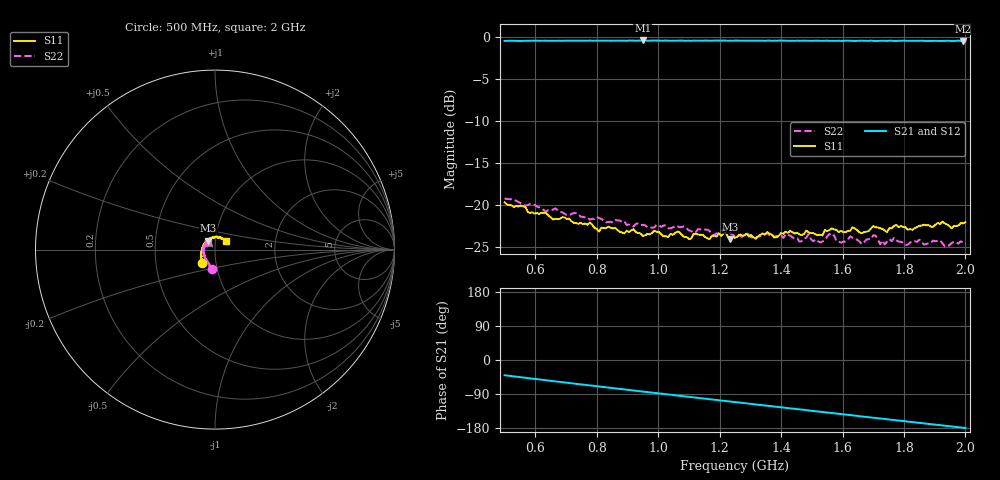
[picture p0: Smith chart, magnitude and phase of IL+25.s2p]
!Agilent Technologies,E8361C,US49010292,A.09.42.06
!Agilent E8361C: A.09.42.06
!Date: Friday, January 10, 2025 01:45:48
!Correction: S11(Full 2 Port(1,2))
!S21(Full 2 Port(1,2))
!S12(Full 2 Port(1,2))
!S22(Full 2 Port(1,2))
!S2P File: Measurements: S11, S21, S12, S22:
# Hz S  dB  R 50
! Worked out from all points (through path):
!   201 points, 500 MHz to 2 GHz, reference 50 ohm
!   highest |S21| = -0.43 dB at 950 MHz (marker M1); lowest = -0.5 dB at 1.992 GHz (marker M2)
!   group delay of S21, straight-line fit = 257 ps
!   lowest |S11| = -24.0 dB at 1.235 GHz (marker M3), VSWR 1.13, Z = 46.1 + j4.63 ohm
!   |S11| at or under -10 dB: start of sweep to end of sweep
!   |S22| runs from -24.9 to -19.2 dB; largest |S21 - S12| = 0.0068
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5e8  -19.67 -132.8  -0.49 -40.3  -0.48 -40.3  -19.23 -97.8
7.55e8  -22.24 -166.1  -0.45 -65.0  -0.46 -65.0  -21.39 -115.4
9.5e8  -23.67 166.5  -0.43 -83.3  -0.45 -83.3  -22.33 -131.7
1.0025e9  -23.20 158.5  -0.44 -88.2  -0.46 -88.1  -22.43 -134.2
1.1e9  -24.02 146.1  -0.46 -97.3  -0.46 -97.2  -23.02 -142.3
1.22e9  -23.29 128.6  -0.44 -108.3  -0.46 -108.3  -22.99 -152.6
1.235e9  -24.05 127.2  -0.45 -109.8  -0.44 -109.6  -23.36 -155.3
1.25e9  -23.88 126.5  -0.44 -110.9  -0.45 -111.2  -23.72 -154.1
1.415e9  -23.14 106.1  -0.45 -126.3  -0.46 -126.2  -23.45 -168.3
1.46e9  -23.50 99.5  -0.47 -130.3  -0.45 -130.4  -24.33 -173.9
1.49e9  -23.24 98.8  -0.48 -133.1  -0.46 -133.1  -23.42 -178.3
1.505e9  -23.31 93.2  -0.46 -134.5  -0.46 -134.5  -24.30 -177.7
1.5575e9  -22.97 87.7  -0.48 -139.3  -0.45 -139.2  -23.42 177.7
1.595e9  -23.06 81.1  -0.48 -142.7  -0.48 -142.8  -24.46 173.3
1.625e9  -23.05 81.6  -0.47 -145.4  -0.48 -145.4  -23.71 172.8
1.6625e9  -23.34 74.9  -0.45 -148.8  -0.46 -149.0  -24.62 166.7
1.7e9  -22.49 72.1  -0.49 -152.4  -0.48 -152.3  -23.59 166.2
1.7225e9  -22.75 67.9  -0.47 -154.4  -0.46 -154.3  -24.66 159.7
1.7525e9  -22.72 66.6  -0.46 -156.9  -0.48 -157.1  -24.04 162.4
1.805e9  -22.62 58.8  -0.46 -161.7  -0.50 -161.9  -24.73 156.2
1.9925e9  -22.18 40.5  -0.51 -178.8  -0.50 -179.0  -24.45 134.8
2e9  -22.02 39.0  -0.50 -179.5  -0.49 -179.4  -24.64 134.4
